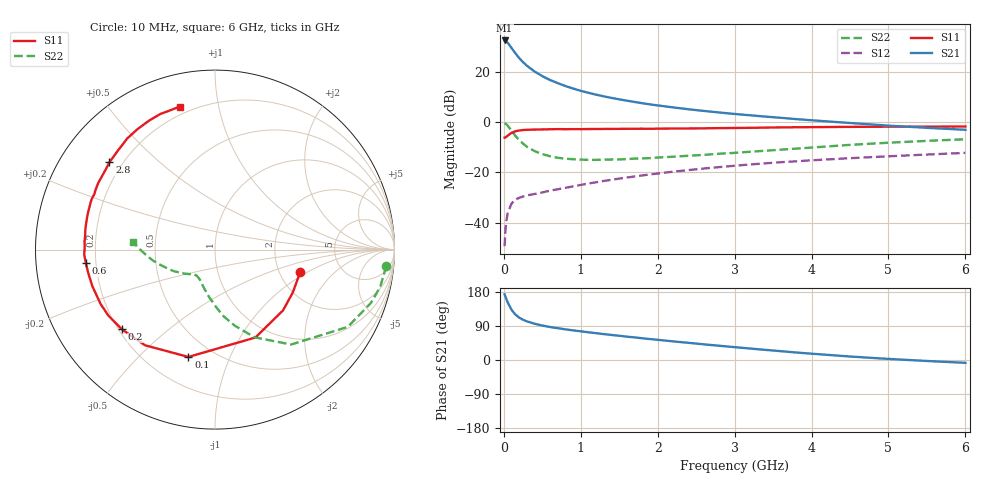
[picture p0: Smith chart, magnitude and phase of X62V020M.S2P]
! SIEMENS Small Signal Semiconductors
! BFP193W
! Si NPN RF Bipolar Junction Transistor in SOT343
! VCE = 2 V  IC = 20 mA
! Common Emitter S-Parameters:  April 1994
# GHz  S  MA  R  50
!  f  S11  S21  S12  S22
! GHz  MAG  ANG  MAG  ANG  MAG  ANG  MAG  ANG
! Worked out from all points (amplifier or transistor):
!   40 points, 10 MHz to 6 GHz, reference 50 ohm
!   highest |S21| = 32.6 dB at 10 MHz (marker M1)
!   |S21| within 3 dB of that: start of sweep to 100.4 MHz
!   unconditionally stable (mu >= 1): 908 MHz to 4.151 GHz
!   at 200 MHz: K = 0.36, MSG = 27.8 dB, |S12| = -30.1 dB
!   at 1.5 GHz: K = 1.12, MAG = 13.7 dB, |S12| = -22.5 dB
!   at 6 GHz: K = 0.93, MSG = 4.6 dB, |S12| = -12.2 dB
!   lowest NFmin = 1.40 dB at 450 MHz
!   S11 on the Smith chart (normalised r, x): 10 MHz: 2.62, -0.84; 100 MHz: 0.37, -0.71; 200 MHz: 0.21, -0.35; 600 MHz: 0.16, -0.05; 2.8 GHz: 0.15, +0.35; 6 GHz: 0.16, +0.77
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0.01  0.4913 -14.4  42.45 173.2  0.0034 85.7  0.9589 -5.5
0.02  0.495 -28.9  42 168.1  0.0068 77.0  0.9434 -12.8
0.03  0.5083 -41.8  41.15 162.5  0.0101 77.0  0.918 -18.9
0.05  0.539 -65.3  38.28 151.9  0.0155 66.7  0.856 -30.2
0.1  0.6161 -103.9  30.11 132.5  0.024 50.9  0.6778 -51.3
0.15  0.6605 -126.2  23.55 119.8  0.0288 43.1  0.5361 -65.7
0.2  0.683 -139.5  18.89 111.8  0.0312 39.6  0.4383 -75.4
0.25  0.6986 -148.2  15.71 106.2  0.0331 37.8  0.3741 -82.7
0.3  0.7057 -154.5  13.31 102.0  0.0349 37.4  0.3241 -88.4
0.4  0.7131 -163.4  10.22 95.6  0.0372 38.2  0.2657 -97.2
0.5  0.7184 -169.6  8.28 90.9  0.04 40.8  0.2315 -103.9
0.6  0.7236 -174.1  6.935 87.1  0.0433 42.7  0.2101 -109.3
0.8  0.726 179.1  5.248 80.9  0.0493 46.5  0.1877 -116.6
1.1  0.7309 171.3  3.856 73.1  0.0601 50.5  0.1778 -124.2
1.3  0.734 166.9  3.269 68.3  0.0677 52.1  0.1792 -127.4
1.6  0.7387 161.0  2.681 61.6  0.0791 53.5  0.184 -131.3
2.2  0.749 150.3  1.973 49.2  0.1034 53.4  0.2053 -139.1
2.8  0.7631 140.4  1.563 37.6  0.1277 51.3  0.2356 -146.4
3.2  0.7732 134.2  1.375 30.3  0.1438 49.1  0.2582 -152.2
4.5  0.8075 116.9  0.964 9.2  0.192 41.0  0.3539 -170.4
5.5  0.8149 108.1  0.773 -2.6  0.2271 34.9  0.425 179.0
6  0.8209 103.8  0.706 -7.5  0.2452 32.1  0.4578 174.9
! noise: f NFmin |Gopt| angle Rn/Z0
0.45  1.4  0.3  160  0.1
0.9  1.45  0.34  172  0.11
1.8  2.2  0.56  -148  0.2
